FUNCTION "ASSE X" : VOID
TITLE =GESTIONE SEGNALI DI STATO E COMANDO DELL'ASSE X
VERSION : 0.1

BEGIN
NETWORK
TITLE =INS./DISIN.1
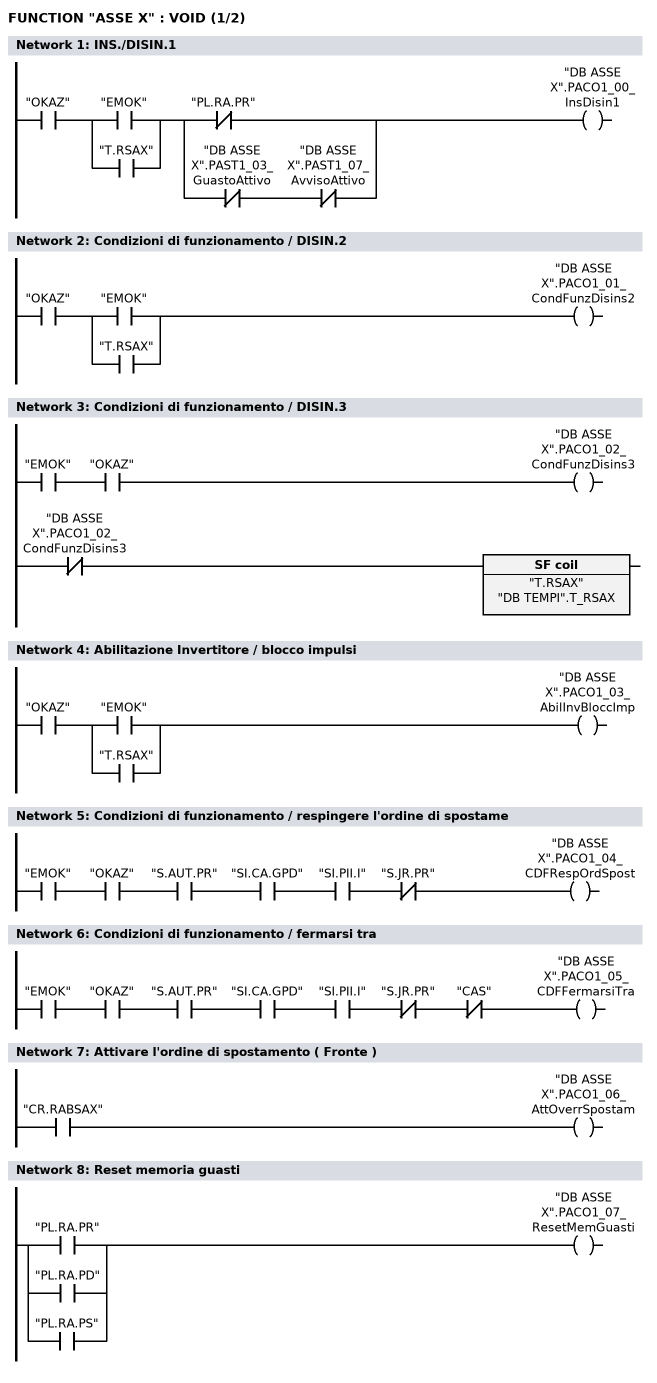
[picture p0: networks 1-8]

      U     "OKAZ";
      U(    ;
      O     "EMOK";
      O     "T.RSAX";
      )     ;
      U(    ;
      UN    "PL.RA.PR";
      O     ;
      UN    "DB ASSE X".PAST1_03_GuastoAttivo;
      UN    "DB ASSE X".PAST1_07_AvvisoAttivo;
      )     ;
      =     "DB ASSE X".PACO1_00_InsDisin1;

NETWORK
TITLE =Condizioni di funzionamento / DISIN.2

      U     "OKAZ";
      U(    ;
      O     "EMOK";
      O     "T.RSAX";
      )     ;
      =     "DB ASSE X".PACO1_01_CondFunzDisins2;

NETWORK
TITLE =Condizioni di funzionamento / DISIN.3

      U     "EMOK";
      U     "OKAZ";
      =     "DB ASSE X".PACO1_02_CondFunzDisins3;
//---------------------------
      UN    "DB ASSE X".PACO1_02_CondFunzDisins3;
      L     "DB TEMPI".T_RSAX;
      SA    "T.RSAX";

NETWORK
TITLE =Abilitazione Invertitore / blocco impulsi

      U     "OKAZ";
      U(    ;
      O     "EMOK";
      O     "T.RSAX";
      )     ;
      =     "DB ASSE X".PACO1_03_AbilInvBloccImp;

NETWORK
TITLE =Condizioni di funzionamento / respingere l'ordine di spostame

      U     "EMOK";
      U     "OKAZ";
      U     "S.AUT.PR";
      U     "SI.CA.GPD";
      U     "SI.PII.I";
      UN    "S.JR.PR";
      =     "DB ASSE X".PACO1_04_CDFRespOrdSpost;

NETWORK
TITLE =Condizioni di funzionamento / fermarsi tra

      U     "EMOK";
      U     "OKAZ";
      U     "S.AUT.PR";
      U     "SI.CA.GPD";
      U     "SI.PII.I";
      UN    "S.JR.PR";
      UN    "CAS";
      =     "DB ASSE X".PACO1_05_CDFFermarsiTra;

NETWORK
TITLE =Attivare l'ordine di spostamento ( Fronte )

      U     "CR.RABSAX";
      =     "DB ASSE X".PACO1_06_AttOverrSpostam;

NETWORK
TITLE =Reset memoria guasti

      U     "PL.RA.PR";
      O     "PL.RA.PD";
      O     "PL.RA.PS";
      =     "DB ASSE X".PACO1_07_ResetMemGuasti;

NETWORK
TITLE =Marcia impulsi 1 INS
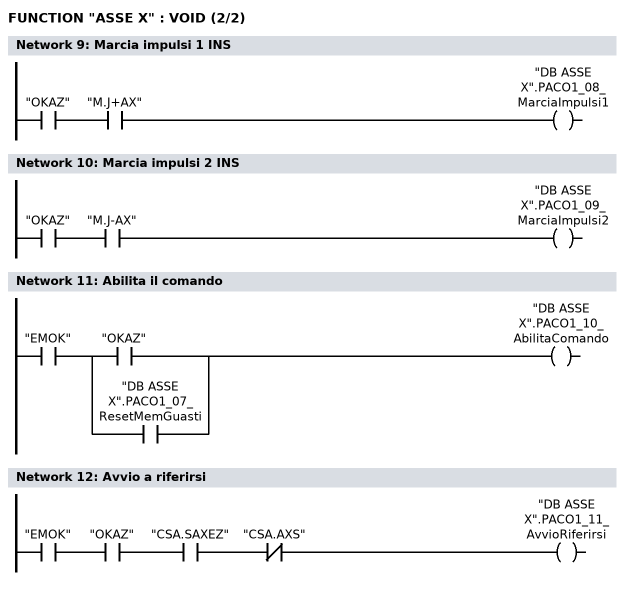
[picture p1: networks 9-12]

      U     "OKAZ";
      U     "M.J+AX";
      =     "DB ASSE X".PACO1_08_MarciaImpulsi1;

NETWORK
TITLE =Marcia impulsi 2 INS

      U     "OKAZ";
      U     "M.J-AX";
      =     "DB ASSE X".PACO1_09_MarciaImpulsi2;

NETWORK
TITLE =Abilita il comando

      U     "EMOK";
      U(    ;
      U     "OKAZ";
      O     ;
      U     "DB ASSE X".PACO1_07_ResetMemGuasti;
      )     ;
      =     "DB ASSE X".PACO1_10_AbilitaComando;

NETWORK
TITLE =Avvio a riferirsi

      U     "EMOK";
      U     "OKAZ";
      U     "CSA.SAXEZ";
      UN    "CSA.AXS";
      =     "DB ASSE X".PACO1_11_AvvioRiferirsi;

NETWORK
TITLE =Cambio del blocco esterno

      CLR   ;
      =     "DB ASSE X".PACO1_13_CambioBloccoExt;

NETWORK
TITLE =Caricamento del numero blocco di spostamento desiderato



NETWORK
TITLE =Funzionamento a seguire

      CLR   ;
      =     "DB ASSE X".POSPACO_00_FunzASeguire;

NETWORK
TITLE =Imposta il punto di riferimento

      CLR   ;
      =     "DB ASSE X".POSPACO_01_ImpostPuntRif;

NETWORK
TITLE =Camma di riferimento

      UN    "FC.ZAX";
      =     "DB ASSE X".POSPACO_02_CammaRiferime;

NETWORK
TITLE =Sensore della battuta fissa

      CLR   ;
      =     "DB ASSE X".POSPACO_03_SensBattFissa;

NETWORK
TITLE =Attivare l'accoppiamento

      CLR   ;
      =     "DB ASSE X".POSPACO_04_AttivAccoppia;

NETWORK
TITLE =Commutazione del blocco di parametri Bit 0

      CLR   ;
      =     "DB ASSE X".PACO2_00_CommBlocParBit1;

NETWORK
TITLE =Commutazione del blocco di parametri Bit 1

      CLR   ;
      =     "DB ASSE X".PACO2_01_CommBlocParBit2;

NETWORK
TITLE =Commutazione del blocco di parametri Bit 2

      CLR   ;
      =     "DB ASSE X".PACO2_02_CommBlocParBit3;

NETWORK
TITLE =Primo filtro nel riferimento di velocita' disinserito

      CLR   ;
      =     "DB ASSE X".PACO2_03_1FiltRifVelDisi;

NETWORK
TITLE =Tempo rampa zero

      CLR   ;
      =     "DB ASSE X".PACO2_04_TempoRampaZero;

NETWORK
TITLE =Blocco dell'integratore nel regolatore di velocita'

      CLR   ;
      =     "DB ASSE X".PACO2_06_BlocIntegrRegV;

NETWORK
TITLE =Scelta dell'asse in parcheggio

      CLR   ;
      =     "DB ASSE X".PACO2_07_SceltaAsseInPar;

NETWORK
TITLE =Tacitare il guasto 608

      U     "OKAZ";
      U     "PL.RA.PR";
      =     "DB ASSE X".PACO2_08_TacitGuasto608;

NETWORK
TITLE =Commutazione dati del motore 1 ingresso

      CLR   ;
      =     "DB ASSE X".PACO2_09_CommDatiMot1Ing;

NETWORK
TITLE =Commutazione dati del motore 2 ingresso

      CLR   ;
      =     "DB ASSE X".PACO2_10_CommDatiMot2Ing;

NETWORK
TITLE =Ha luogo la ommutazione del motore

      CLR   ;
      =     "DB ASSE X".PACO2_11_CommutazMotore;

NETWORK
TITLE =OVERRIDE

      U     "M.MAN";
      UN    "P.JR.PR";
      SPBN  E001;
      L     "DB DATI".OVERRIDE_JOG;
      T     "DB ASSE X".OVERRIDE;
      T     "DB DATI".OVERRIDE_ATTIVO;
E001: NOP   0;
      U     "M.MAN";
      U     "P.JR.PR";
      SPBN  E002;
      L     "DB DATI".OVERRIDE_JOG;
      L     2;
      *I    ;
      T     "DB ASSE X".OVERRIDE;
      T     "DB DATI".OVERRIDE_ATTIVO;
E002: NOP   0;
      UN    "M.MAN";
      SPBN  E003;
      L     "DB DATI".OVERRIDE_AUT;
      T     "DB ASSE X".OVERRIDE;
      T     "DB DATI".OVERRIDE_ATTIVO;
E003: NOP   0;

NETWORK
TITLE =Riduzione percentuale del limite di coppia

      L     0;
      T     "DB ASSE X".MOMRID;

NETWORK
TITLE =Caricamento quote

      U     "ANSD";
      UN    "CQAX.IC";
      S     "CQAX.IC";
      S     "CQAX.Q1";
//============================ QUOTA 1
      U     "CQAX.Q1";
      SPBN  END1;
      L     W#16#8051;
      T     "DB ASSE X".PKE_Scrittura;
      L     W#16#1;
      T     "DB ASSE X".IND_Scrittura;
      L     "DB QUOTE".X_ATTESA;
      T     DB121.DBD    4;
//----------------------------
      U(    ;
      L     "DB ASSE X".PKE_Lettura;
      L     W#16#5051;
      ==I   ;
      )     ;
      U(    ;
      L     "DB ASSE X".IND_Lettura;
      L     W#16#1;
      ==I   ;
      )     ;
      R     "CQAX.Q1";
      S     "CQAX.Q2";
END1: NOP   0;
//============================ QUOTA 2
      U     "CQAX.Q2";
      SPBN  END2;
      L     W#16#8051;
      T     "DB ASSE X".PKE_Scrittura;
      L     W#16#2;
      T     "DB ASSE X".IND_Scrittura;
      L     "DB QUOTE".X_FUORI_INGOMBRO;
      T     DB121.DBD    4;
//----------------------------
      U(    ;
      L     "DB ASSE X".PKE_Lettura;
      L     W#16#5051;
      ==I   ;
      )     ;
      U(    ;
      L     "DB ASSE X".IND_Lettura;
      L     W#16#2;
      ==I   ;
      )     ;
      R     "CQAX.Q2";
      S     "CQAX.Q3";
END2: NOP   0;
//============================ QUOTA 3
      U     "CQAX.Q3";
      SPBN  END3;
      L     W#16#8051;
      T     "DB ASSE X".PKE_Scrittura;
      L     W#16#3;
      T     "DB ASSE X".IND_Scrittura;
      L     "DB QUOTE".X_DEPOSITO;
      T     DB121.DBD    4;
//----------------------------
      U(    ;
      L     "DB ASSE X".PKE_Lettura;
      L     W#16#5051;
      ==I   ;
      )     ;
      U(    ;
      L     "DB ASSE X".IND_Lettura;
      L     W#16#3;
      ==I   ;
      )     ;
      R     "CQAX.Q3";
      S     "CQAX.V1";
END3: NOP   0;
//============================ VELOCITA' 1
      U     "CQAX.V1";
      SPBN  END4;
      L     W#16#8052;
      T     "DB ASSE X".PKE_Scrittura;
      L     W#16#1;
      T     "DB ASSE X".IND_Scrittura;
      L     "DB QUOTE".VELOCITA_X;
      T     DB121.DBD    4;
//----------------------------
      U(    ;
      L     "DB ASSE X".PKE_Lettura;
      L     W#16#5052;
      ==I   ;
      )     ;
      U(    ;
      L     "DB ASSE X".IND_Lettura;
      L     W#16#1;
      ==I   ;
      )     ;
      R     "CQAX.V1";
      S     "CQAX.V2";
END4: NOP   0;
//============================ VELOCITA' 2
      U     "CQAX.V2";
      SPBN  END5;
      L     W#16#8052;
      T     "DB ASSE X".PKE_Scrittura;
      L     W#16#2;
      T     "DB ASSE X".IND_Scrittura;
      L     "DB QUOTE".VELOCITA_X;
      T     DB121.DBD    4;
//----------------------------
      U(    ;
      L     "DB ASSE X".PKE_Lettura;
      L     W#16#5052;
      ==I   ;
      )     ;
      U(    ;
      L     "DB ASSE X".IND_Lettura;
      L     W#16#2;
      ==I   ;
      )     ;
      R     "CQAX.V2";
      S     "CQAX.V3";
END5: NOP   0;
//============================ VELOCITA' 3
      U     "CQAX.V3";
      SPBN  END6;
      L     W#16#8052;
      T     "DB ASSE X".PKE_Scrittura;
      L     W#16#3;
      T     "DB ASSE X".IND_Scrittura;
      L     "DB QUOTE".VELOCITA_X;
      T     DB121.DBD    4;
//----------------------------
      U(    ;
      L     "DB ASSE X".PKE_Lettura;
      L     W#16#5052;
      ==I   ;
      )     ;
      U(    ;
      L     "DB ASSE X".IND_Lettura;
      L     W#16#3;
      ==I   ;
      )     ;
      R     "CQAX.V3";
      S     "CQAX.CT";
END6: NOP   0;
      U     "CQAX.CT";
      UN    "ANSD";
      R     "CQAX.CT";
      R     "CQAX.IC";

NETWORK
TITLE =LETTURA ALLARMI

      U     "DB ASSE X".PAST1_03_GuastoAttivo;

END_FUNCTION

